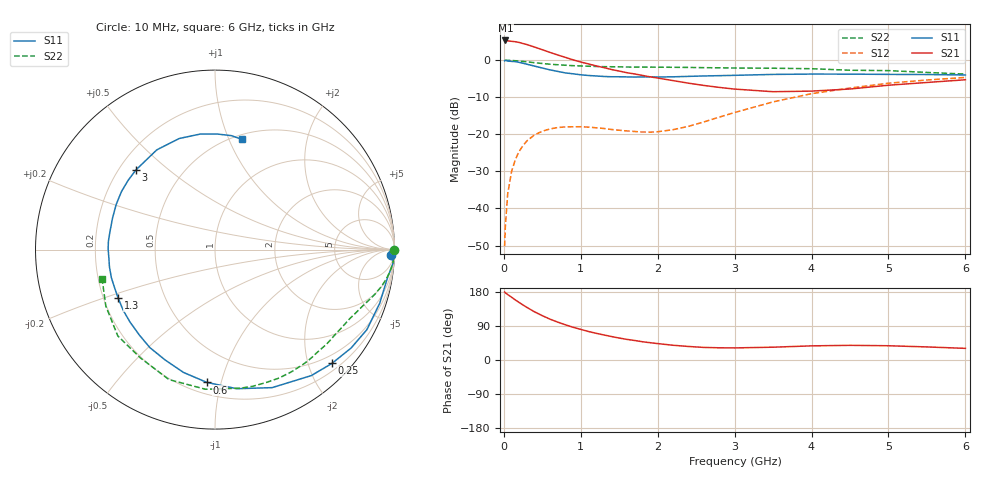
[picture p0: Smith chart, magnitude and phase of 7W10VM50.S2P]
! Infineon Technologies  Discrete & RF Semiconductors
! BFS17W
! Si NPN RF Bipolar Junction Transistor in SOT323
! VCE = 10 V  IC = 0.5 mA
! Common Emitter S-Parameters:  August  1999
# GHz  S  MA  R  50
!  f  S11  S21  S12  S22
! GHz  MAG  ANG  MAG  ANG  MAG  ANG  MAG  ANG
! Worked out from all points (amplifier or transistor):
!   36 points, 10 MHz to 6 GHz, reference 50 ohm
!   highest |S21| = 5.3 dB at 20 MHz (marker M1)
!   |S21| within 3 dB of that: start of sweep to 568.8 MHz
!   unconditionally stable (mu >= 1): 1.258 GHz to end of sweep
!   at 250 MHz: K = 0.21, MSG = 13.8 dB, |S12| = -23.0 dB
!   at 1.4 GHz: K = 1.12, MAG = 5.9 dB, |S12| = -18.7 dB
!   at 6 GHz: K = 1.08, MAG = -2.1 dB, |S12| = -4.6 dB
!   S11 on the Smith chart (normalised r, x): 10 MHz: 29, -45; 250 MHz: 0.33, -2.42; 600 MHz: 0.27, -0.90; 1.3 GHz: 0.26, -0.22; 3 GHz: 0.27, +0.39; 6 GHz: 0.55, +1.12
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0.01  0.9798 -1.8  1.825 179.3  0.0031 88.8  0.9999 0.0
0.02  0.9967 -4.0  1.848 177.2  0.0058 84.3  0.9992 -0.9
0.05  0.974 -9.2  1.827 172.7  0.0157 85.3  0.9972 -2.3
0.1  0.9652 -18.0  1.8 165.8  0.0314 79.1  0.9933 -4.5
0.15  0.9567 -27.8  1.776 158.4  0.0459 73.7  0.9841 -6.7
0.25  0.9093 -44.2  1.678 145.1  0.0707 63.9  0.9628 -10.5
0.3  0.8835 -52.6  1.627 138.8  0.0816 59.8  0.951 -12.3
0.4  0.8324 -67.5  1.504 127.0  0.0986 52.1  0.926 -15.5
0.5  0.7845 -81.1  1.387 117.0  0.1102 45.8  0.9032 -18.1
0.6  0.7413 -93.5  1.274 107.8  0.1183 40.7  0.8837 -20.5
0.8  0.6748 -114.3  1.093 92.9  0.1261 33.6  0.8554 -25.0
1.1  0.6222 -139.6  0.891 75.2  0.1252 28.0  0.8294 -31.4
1.3  0.6034 -153.4  0.795 66.1  0.12 27.7  0.8188 -35.9
1.6  0.5958 -170.8  0.678 54.4  0.1112 31.8  0.8102 -42.8
2.2  0.5973 162.9  0.531 38.9  0.1156 55.1  0.803 -58.1
3  0.6254 134.8  0.408 31.9  0.1971 73.2  0.7851 -79.5
3.5  0.6434 120.3  0.376 33.8  0.2742 72.0  0.7799 -93.9
4  0.6503 107.9  0.383 37.3  0.3538 66.3  0.7682 -109.5
4.5  0.6491 97.2  0.409 38.7  0.4214 59.0  0.7327 -124.5
5  0.644 88.9  0.46 37.6  0.4897 51.7  0.7243 -138.4
5.5  0.6414 81.8  0.501 34.5  0.541 44.2  0.6846 -152.7
6  0.6322 76.2  0.545 30.7  0.5857 37.3  0.65 -165.3
